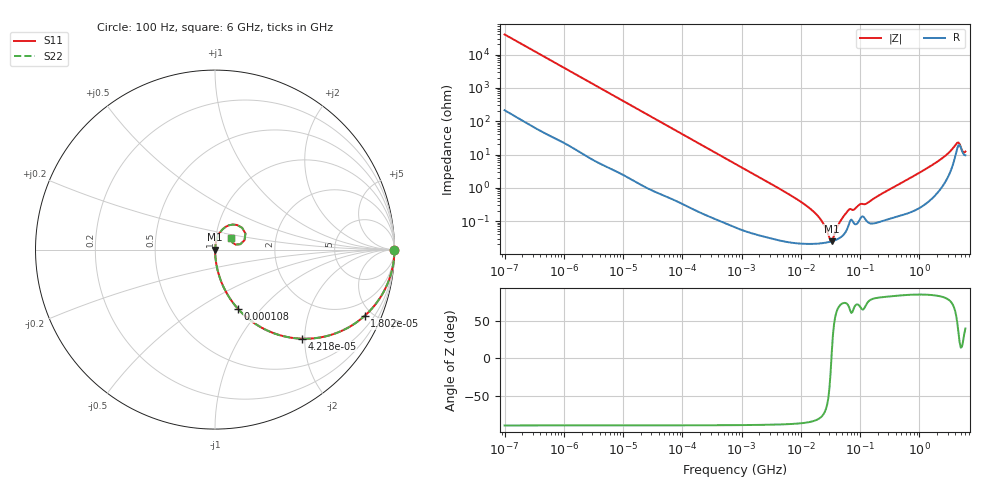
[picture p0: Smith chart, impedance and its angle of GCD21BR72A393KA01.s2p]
!Murata Part Number: GCD21BR72A393KA01
!These Parameters are Measured in Series Mode Connection
!Data Generated on Mar 13, 2026
!  o--ll--o
!Port1  Port2
!  o------o
!Operation Temp=25[degC], DC Bias Voltage=0[V]
!Freq. Start=100[Hz] Stop=6[GHz] 401[Steps]
# Hz S RI R 50
!Freq.(Hz) S11(Real) S11(Imag) S21(Real) S21(Imag) S12(Real) S12(Imag) S22(Real) S22(Imag)
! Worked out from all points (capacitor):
!   401 points, 100 Hz to 6 GHz, reference 50 ohm
!   read as one part in series: C = 39.8 nF near 109 Hz
!   lowest |Z| = 25.2 mohm at 33.3 MHz (marker M1)
!   series resonance near 32.87 MHz, so ESL is about 590 pH
!   S11 on the Smith chart (normalised r, x): 100 Hz: open; 18.02 kHz: 1.03, -4.52; 42.18 kHz: 1.01, -1.93; 108 kHz: 1.01, -0.76; 6 GHz: 1.19, +0.16
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100  1 -0.0025  1.96e-05 0.0025  1.96e-05 0.0025  1 -0.0025
2008  0.9973 -0.0496  0.00273 0.0496  0.00273 0.0496  0.9973 -0.0496
8047  0.9611 -0.1905  0.0389 0.1905  0.0389 0.1905  0.9611 -0.1905
18016  0.8346 -0.3685  0.1654 0.3685  0.1654 0.3685  0.8346 -0.3685
40335  0.5057 -0.4966  0.4943 0.4966  0.4943 0.4966  0.5057 -0.4966
42182  0.4835 -0.4964  0.5165 0.4964  0.5165 0.4964  0.4835 -0.4964
108014  0.1279 -0.3299  0.8721 0.3299  0.8721 0.3299  0.1279 -0.3299
276587  0.023 -0.1452  0.977 0.1452  0.977 0.1452  0.023 -0.1452
774597  0.00349 -0.0532  0.9965 0.0532  0.9965 0.0532  0.00349 -0.0532
6644369  0.000266 -0.00606  0.9997 0.00606  0.9997 0.00606  0.000266 -0.00606
1.555665e7  0.000213 -0.0021  0.9998 0.0021  0.9998 0.0021  0.000213 -0.0021
2.225763e7  0.000218 -0.00103  0.9998 0.00103  0.9998 0.00103  0.000218 -0.00103
3.045065e7  0.000239 -0.000198  0.9998 0.000198  0.9998 0.000198  0.000239 -0.000198
3.330331e7  0.000249 3.47e-05  0.9998 -3.47e-05  0.9998 -3.47e-05  0.000249 3.47e-05
4.556224e7  0.000317 0.000888  0.9997 -0.000888  0.9997 -0.000888  0.000317 0.000888
6.233367e7  0.000664 0.00194  0.9993 -0.00194  0.9993 -0.00194  0.000664 0.00194
1.334425e8  0.000965 0.00339  0.999 -0.00339  0.999 -0.00339  0.000965 0.00339
3.124326e8  0.00125 0.00883  0.9988 -0.00883  0.9988 -0.00883  0.00125 0.00883
1.873145e9  0.00905 0.0548  0.9909 -0.0548  0.9909 -0.0548  0.00905 0.0548
4.193612e9  0.1238 0.137  0.8762 -0.137  0.8762 -0.137  0.1238 0.137
4.586474e9  0.1694 0.0896  0.8306 -0.0896  0.8306 -0.0896  0.1694 0.0896
6e9  0.091 0.0651  0.909 -0.0651  0.909 -0.0651  0.091 0.0651
